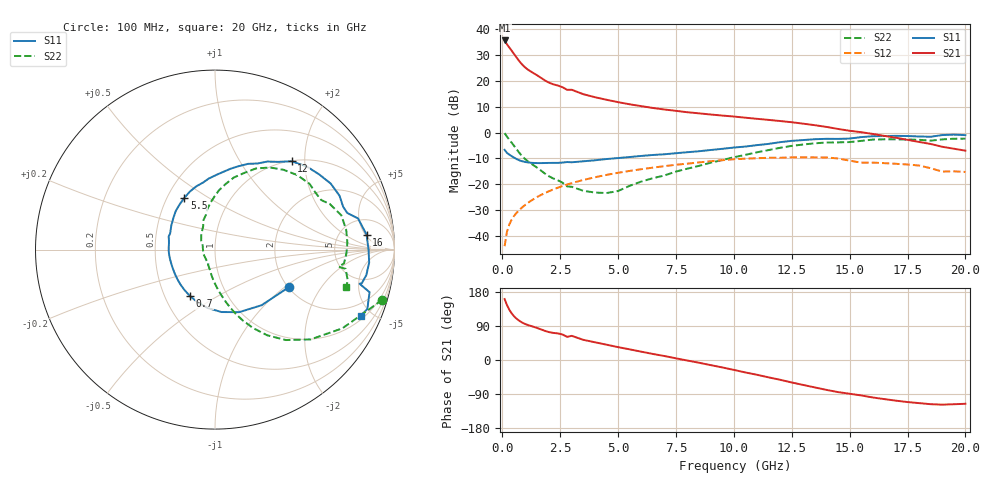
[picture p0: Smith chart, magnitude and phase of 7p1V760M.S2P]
! Infineon Technologies  Discrete & RF Semiconductors
! bfp620
! VCE =  1.7 V,  IC =  60 mA
! Common Emitter S-Parameters:  Sep 2002
# GHz  S  MA  R  50
!  f  S11  S21  S12  S22
! GHz  MAG  ANG  MAG  ANG  MAG  ANG  MAG  ANG
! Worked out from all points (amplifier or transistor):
!   59 points, 100 MHz to 20 GHz, reference 50 ohm
!   highest |S21| = 35.7 dB at 100 MHz (marker M1)
!   |S21| within 3 dB of that: start of sweep to 324.5 MHz
!   unconditionally stable (mu >= 1): 2.634 GHz to 2.972 GHz; 3.06 GHz to 9.848 GHz; 17.18 GHz to end of sweep
!   at 1 GHz: K = 0.87, MSG = 26.5 dB, |S12| = -28.0 dB
!   at 5.5 GHz: K = 1.04, MAG = 11.7 dB, |S12| = -14.9 dB
!   at 20 GHz: K = 1.28, MAG = 0.9 dB, |S12| = -15.2 dB
!   S11 on the Smith chart (normalised r, x): 100 MHz: 2.03, -1.07; 700 MHz: 0.67, -0.38; 5.5 GHz: 0.61, +0.40; 12 GHz: 1.01, +1.72; 16 GHz: 9, +5; 20 GHz: 1.20, -4.30
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0.1  0.4629 -26.7  60.69 160.8  0.0063 81.3  0.9738 -16.7
0.2  0.4042 -50.1  51.25 145.1  0.0119 73.5  0.8346 -31.7
0.3  0.3736 -68.9  44.45 132.9  0.0165 70.4  0.7309 -43.2
0.4  0.3497 -84.1  38.69 123.4  0.0204 68.5  0.6405 -51.9
0.5  0.3281 -97.0  33.55 116.0  0.024 67.3  0.5585 -58.7
0.6  0.3093 -108.2  29.05 109.9  0.0273 66.5  0.4858 -64.1
0.7  0.2942 -118.1  25.27 105.0  0.0305 65.9  0.424 -68.6
0.8  0.2828 -126.6  22.21 100.9  0.0337 65.4  0.3736 -72.3
0.9  0.2744 -133.8  19.84 97.5  0.0368 65.0  0.3337 -75.3
1.1  0.264 -144.9  16.62 92.4  0.0432 64.4  0.2782 -80.0
1.9  0.2573 -175.0  9.855 75.7  0.0692 59.8  0.1537 -95.9
2.8  0.2685 164.0  6.715 61.1  0.0984 52.5  0.0906 -115.8
3  0.2654 160.5  6.732 63.7  0.1048 50.6  0.089 -114.4
3.5  0.2775 151.4  5.524 53.2  0.1207 45.9  0.0743 -132.2
5.5  0.3352 120.6  3.522 28.1  0.1804 26.6  0.0928 146.2
7  0.3792 100.2  2.793 10.5  0.2232 11.8  0.1473 116.4
10.5  0.5351 63.7  1.937 -32.9  0.3119 -27.9  0.37 80.8
12  0.6515 49.1  1.671 -52.2  0.3242 -45.7  0.5067 63.2
13.5  0.7423 29.7  1.387 -72.4  0.3301 -64.5  0.6183 42.2
16  0.8486 5.6  0.94 -98.9  0.2612 -88.4  0.7298 15.1
17  0.862 -4.8  0.793 -107.3  0.2482 -96.3  0.7386 3.0
20  0.8911 -24.4  0.446 -115.6  0.1728 -105.9  0.7612 -15.9
